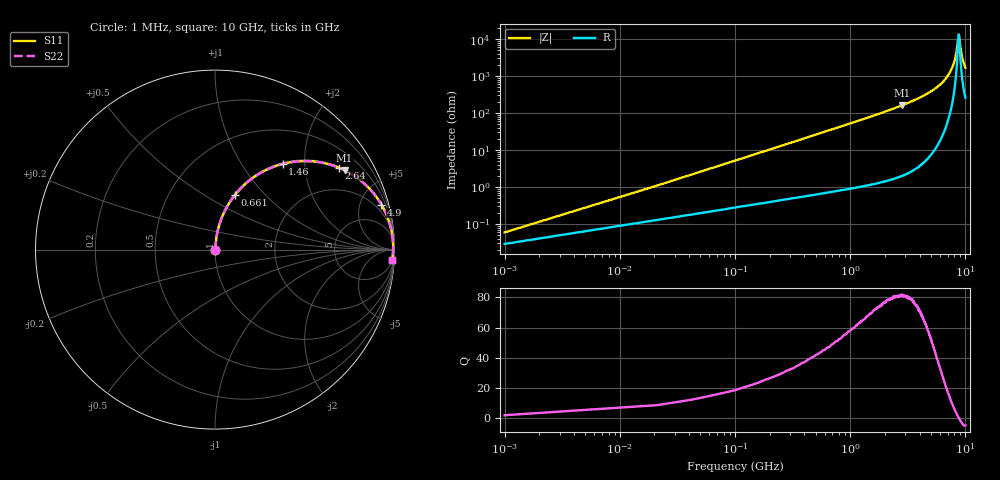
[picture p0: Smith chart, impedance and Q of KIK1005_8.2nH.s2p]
!version-3
!date-01.2023
!Series
# MHz S RI R 50
!Freq ReS11 ImS11 ReS21 ImS21 ReS12 ImS12 ReS22 ImS22
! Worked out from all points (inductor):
!   501 points, 1 MHz to 10 GHz, reference 50 ohm
!   read as one part in series: L = 8.2 nH near 41 MHz
!   highest Q = 81.2 at 2.82 GHz (marker M1), where L = 9.15 nH
!   self-resonance near 8.76 GHz
!   S11 on the Smith chart (normalised r, x): 1 MHz: 1.00, +0.00; 661 MHz: 1.01, +0.69; 1.46 GHz: 1.02, +1.55; 2.64 GHz: 1.04, +2.99; 4.9 GHz: 1.13, +7.35; 10 GHz: 6, -33
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1  0.000277 0.000515  0.9997 -0.000515  0.9997 -0.000515  0.000277 0.000515
61  0.00314 0.0313  0.9969 -0.0313  0.9969 -0.0313  0.00314 0.0313
101  0.00545 0.0516  0.9945 -0.0516  0.9945 -0.0516  0.00545 0.0516
141  0.00848 0.0718  0.9915 -0.0718  0.9915 -0.0718  0.00848 0.0718
221  0.0168 0.1116  0.9832 -0.1116  0.9832 -0.1116  0.0168 0.1116
341  0.0347 0.169  0.9653 -0.169  0.9653 -0.169  0.0347 0.169
661  0.1101 0.3026  0.8899 -0.3026  0.8899 -0.3026  0.1101 0.3026
1460  0.3766 0.4773  0.6234 -0.4773  0.6234 -0.4773  0.3766 0.4773
1680  0.4478 0.4904  0.5522 -0.4904  0.5522 -0.4904  0.4478 0.4904
2640  0.6892 0.4567  0.3108 -0.4567  0.3108 -0.4567  0.6892 0.4567
2820  0.722 0.4419  0.278 -0.4419  0.278 -0.4419  0.722 0.4419
3340  0.7992 0.3943  0.2008 -0.3943  0.2008 -0.3943  0.7992 0.3943
4900  0.9271 0.2511  0.0729 -0.2511  0.0729 -0.2511  0.9271 0.2511
5020  0.9328 0.241  0.0672 -0.241  0.0672 -0.241  0.9328 0.241
6680  0.9802 0.1186  0.0198 -0.1186  0.0198 -0.1186  0.9802 0.1186
7700  0.9905 0.0566  0.00952 -0.0566  0.00952 -0.0566  0.9905 0.0566
8060  0.992 0.0366  0.00799 -0.0366  0.00799 -0.0366  0.992 0.0366
8340  0.9926 0.0217  0.00741 -0.0217  0.00741 -0.0217  0.9926 0.0217
8700  0.9926 0.00326  0.00735 -0.00326  0.00735 -0.00326  0.9926 0.00326
8780  0.9926 -0.000728  0.00743 0.000728  0.00743 0.000728  0.9926 -0.000728
9300  0.9913 -0.0258  0.00875 0.0258  0.00875 0.0258  0.9913 -0.0258
10000  0.9877 -0.0572  0.0123 0.0572  0.0123 0.0572  0.9877 -0.0572
